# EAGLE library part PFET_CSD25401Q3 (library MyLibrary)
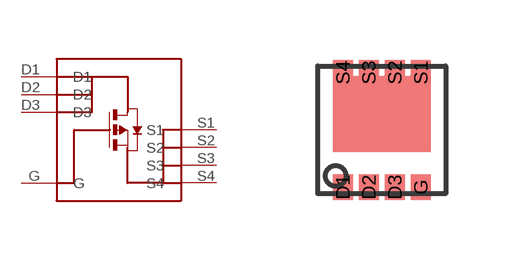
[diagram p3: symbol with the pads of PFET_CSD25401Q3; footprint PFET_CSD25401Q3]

Designator prefix -

## PFET_CSD25401Q3  [PFET_CSD25401Q3]
D1  D1
D2  D2
D3  D3
G  G
S1  S1
S2  S2
S3  S3
S4  S4

## Footprint PFET_CSD25401Q3 (pad centres in mm)
smd 0.5 x 0.63: D1 -0.975,-1.435; D2 -0.325,-1.435; D3 0.325,-1.435; G 0.975,-1.435; S1 0.975,1.435; S2 0.325,1.435; S3 -0.325,1.435; S4 -0.975,1.435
